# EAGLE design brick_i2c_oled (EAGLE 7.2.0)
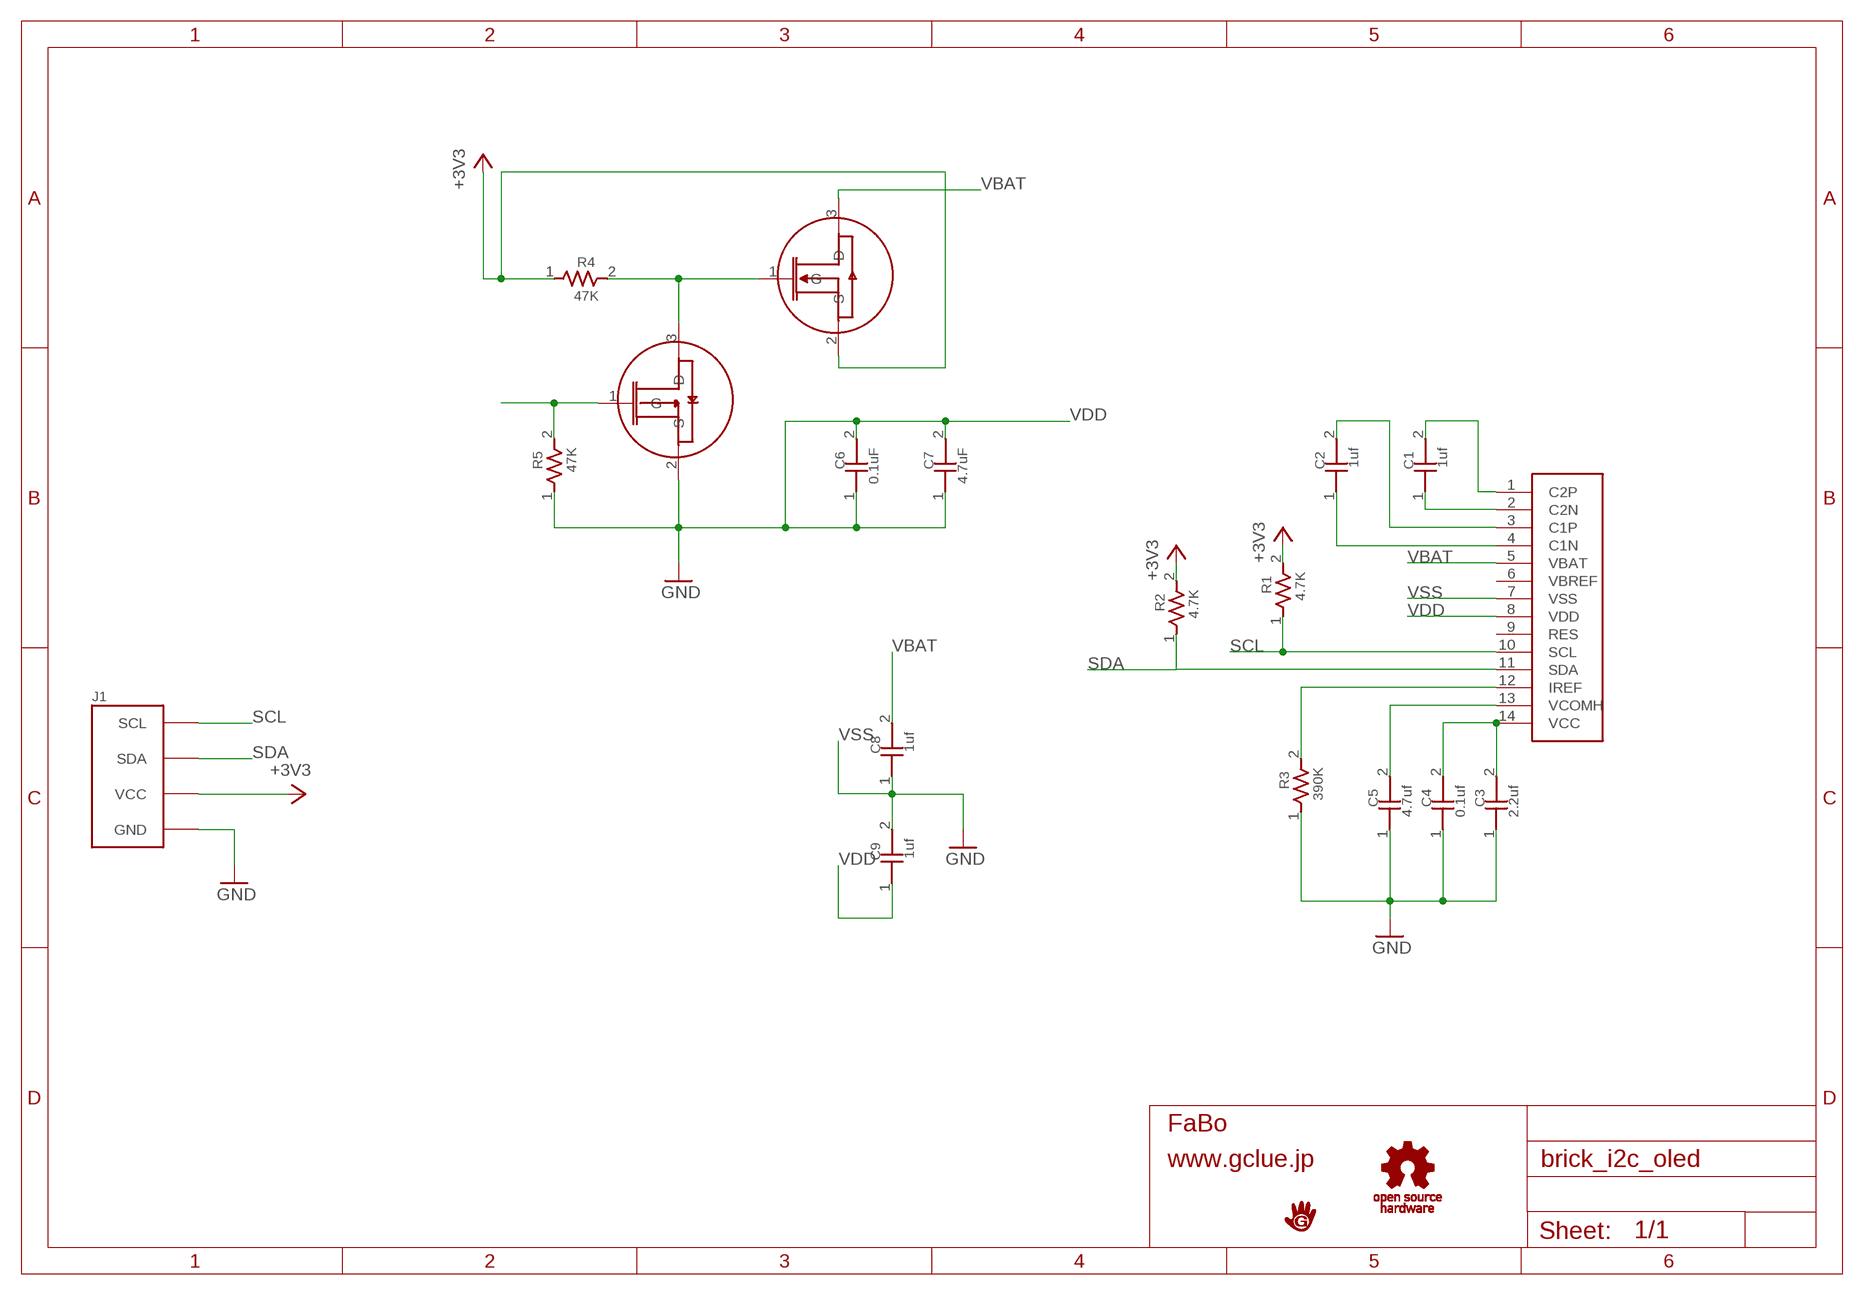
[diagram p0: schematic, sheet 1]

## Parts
C1  1uf  CAPACITOR0603  [0603]
C2  1uf  CAPACITOR0603  [0603]
C3  2.2uf  CAPACITOR0603  [0603]
C4  0.1uf  CAPACITOR0603  [0603]
C5  4.7uf  CAPACITOR0603  [0603]
C6  0.1uF  CAPACITOR0603  [0603]
C7  4.7uF  CAPACITOR0603  [0603]
C8  1uf  CAPACITOR0603  [0603]
C9  1uf  CAPACITOR0603  [0603]
J1  BRICK_I2C  [BRICK_I2C]
R1  4.7K  RESISTOR0603  [0603]
R2  4.7K  RESISTOR0603  [0603]
R3  390K  RESISTOR0603  [0603]
R4  47K  RESISTOR0603  [0603]
R5  47K  RESISTOR0603  [0603]
U$1  LOGO_GCLUE-M  [LOGO_GCLUE_M]
U$2  EASTRISING-ER-OLED0.49-1  [EASTRISING-ER-OLED0.49-1]
U$4  FAIRCHILD-FDN335  [SOT23]
U$5  FAIRCHILD-FDN338  [SOT23]
U$6  LOGO_OSHW_T-M  [LOGO_OSHW_T_M]

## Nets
+3V3: J1.VCC R1.2 R2.2 R4.1 U$4.2(S)
GND: C3.1 C4.1 C5.1 J1.GND R3.1
N$1: C1.2 U$2.1(C2P)
N$2: C1.1 U$2.2(C2N)
N$3: C2.2 U$2.3(C1P)
N$4: C2.1 U$2.4(C1N)
N$5: R5.2 U$5.1(G)
N$6: R3.2 U$2.12(IREF)
N$7: C5.2 U$2.13(VCOMH)
N$8: R4.2 U$4.1(G) U$5.3(D)
SCL: J1.SCL R1.1 U$2.10(SCL)
SDA: J1.SDA R2.1 U$2.11(SDA)
VBAT: C8.2 U$2.5(VBAT) U$4.3(D)
VCC: C3.2 C4.2 U$2.14(VCC)
VDD: C6.1 C6.2 C7.1 C7.2 C9.1 R5.1 U$2.8(VDD) U$5.2(S) ; supply symbol labelled GND
VSS: C8.1 C9.2 U$2.7(VSS) ; supply symbol labelled GND
Unconnected: U$2.6(VBREF) U$2.9(RES)

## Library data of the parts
C1-C9 = GClue-Capacitor:CAPACITOR
J1 = gclue:BRICK_I2C: FaBo Brick 4pin(I2C)
R1-R5 = GClue-Resistors:RESISTOR
U$1 = gclue:LOGO_GCLUE
U$2 = gclueParts:EASTRISING-ER-OLED0.49-1
U$4 = gclueParts:FAIRCHILD-FDN335
U$5 = gclueParts:FAIRCHILD-FDN338
U$6 = gclue:LOGO_OSHW_T

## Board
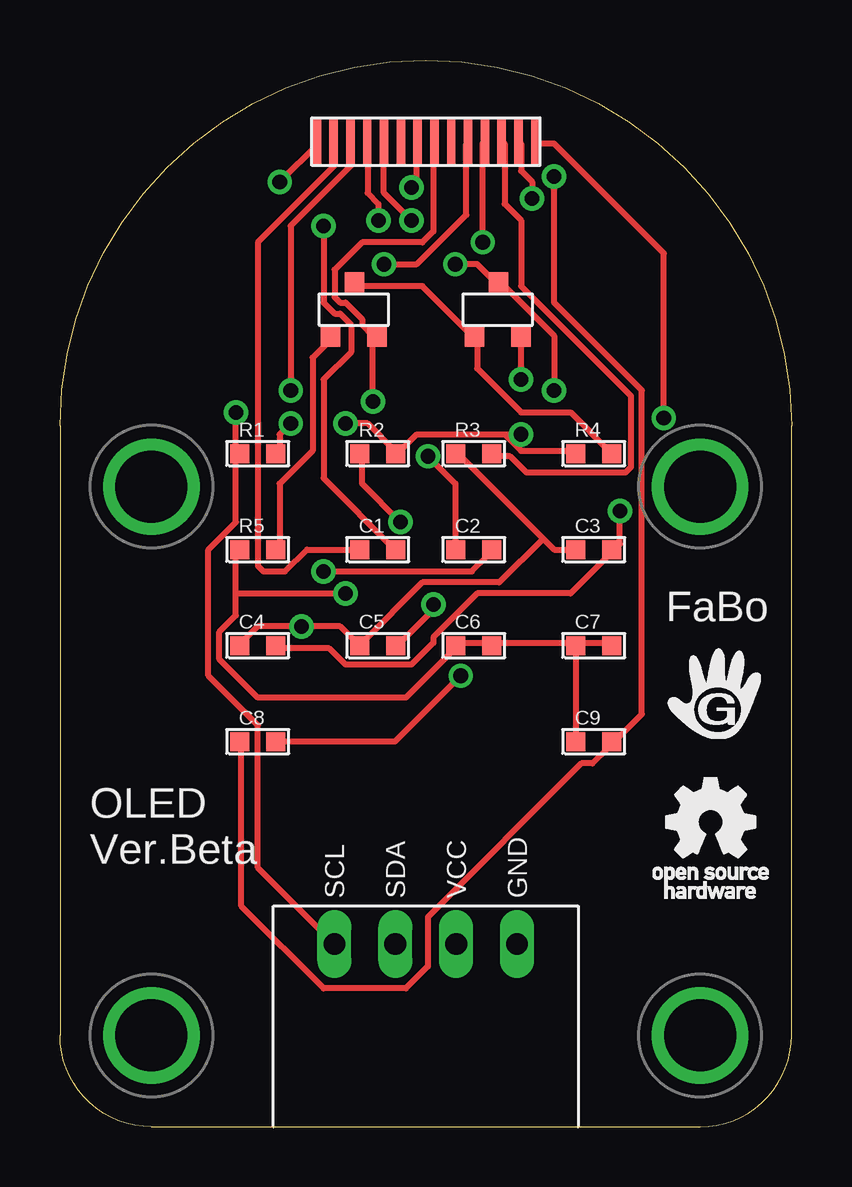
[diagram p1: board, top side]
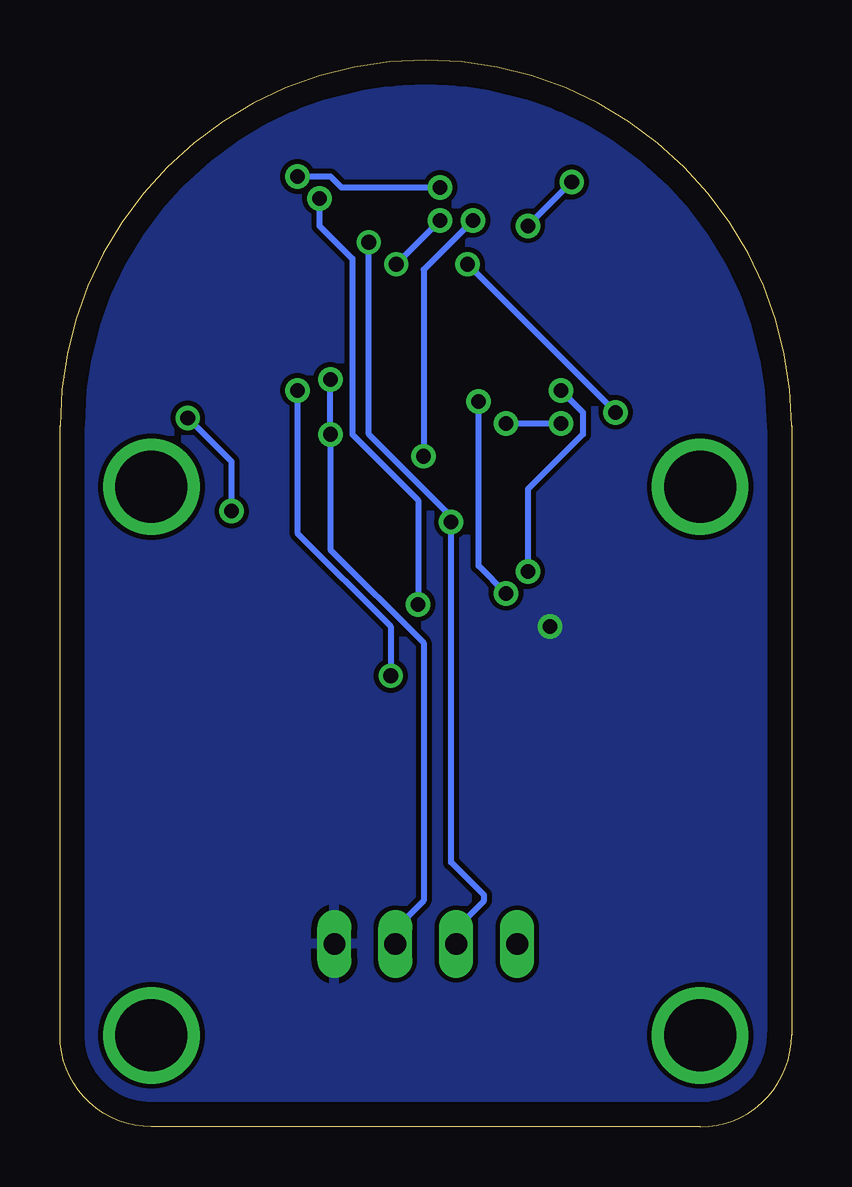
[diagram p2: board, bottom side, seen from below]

Size 30.48 x 44.45 mm. Coordinates in mm from the lower left corner, seen from the top.
Copper layers (1*16): Top 0.035mm / dielectric 1.5mm / Bottom 0.035mm
Design rules "default": minimum track width 10mil, minimum drill 24mil, track to track 8mil, track to pad 8mil, pad to pad 8mil, via to via 8mil, smd to smd 8mil, copper to edge 40mil, drill to drill 8mil, minimum pad ring 10mil, minimum via ring 8mil, stop-mask expansion 4mil, vias tented up to drill 0mil, thermal gap 10mil

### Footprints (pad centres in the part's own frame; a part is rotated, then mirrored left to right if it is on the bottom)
0603 = smd 0.8 x 0.8: 1 -0.75,0; 2 0.75,0
BRICK_I2C = drill 0.9 long: GND 3.81,-11.43; SCL -3.81,-11.43; SDA -1.27,-11.43; VCC 1.27,-11.43 | drill 3 pad 3.81: P$5 -11.43,7.62; P$6 11.43,7.62; P$7 -11.43,-15.24; P$8 11.43,-15.24
EASTRISING-ER-OLED0.49-1 = smd 0.35 x 2: 1 -4.54,0; 2 -3.84,0; 3 -3.14,0; 4 -2.44,0; 5 -1.74,0; 6 -1.04,0; 7 -0.34,0; 8 0.36,0; 9 1.06,0; 10 1.76,0; 11 2.46,0; 12 3.16,0; 13 3.86,0; 14 4.56,0
SOT23 = smd 0.8 x 0.9: 1 -0.97,-1.1; 2 0.97,-1.1; 3 0.03,1.1

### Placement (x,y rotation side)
C1  13.24,24.05 0 top
C2  17.24,24.05 0 top
C3  22.24,24.05 0 top
C4  8.24,20.05 0 top
C5  13.24,20.05 0 top
C6  17.24,20.05 0 top
C7  22.24,20.05 0 top
C8  8.24,16.05 0 top
C9  22.24,16.05 0 top
J1  15.24,19.05 0 top
R1  8.24,28.05 0 top
R2  13.24,28.05 0 top
R3  17.24,28.05 0 top
R4  22.24,28.05 0 top
R5  8.24,24.05 0 top
U$1  27.24,18.05 0 top
U$2  15.24,41.05 0 top
U$4  18.24,34.05 0 top
U$5  12.24,34.05 0 top
U$6  27.24,12.05 0 top

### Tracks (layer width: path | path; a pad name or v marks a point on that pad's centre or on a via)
+3V3  (via drill 0.61)
  Top 0.254: v9.61,29.31 9.15,28.85 9.15,28.17 R1.2 | v11.9,29.31 12.81,29.31 13.96,28.17 R2.2 14.19,28.17 14.87,28.85 18.53,28.85 | 18.53,28.85 19.21,28.17 21.27,28.17 R4.1 | v19.21,31.14 19.21,32.74 U$4.2 | 18.53,28.85 v19.21,28.85
  Bottom 0.254: v11.9,29.31 v9.61,29.31 | v19.21,31.14 v19.21,28.85 19.21,24.05 15.33,20.17 15.33,9.42 16.47,8.28 16.47,7.82 J1.VCC
GND  (via drill 0.61)
  Top 0.254: C4.1 7.56,20.17 8.24,20.85 v10.07,20.85 11.67,20.85 12.36,20.17 C5.1 12.58,20.17 15.1,22.68 18.3,22.68 20.13,24.51 | 20.13,24.51 16.7,27.94 R3.1 | 20.13,24.51 20.59,24.05 21.27,24.05 C3.1
  pour Bottom: 0.24,0.05 30.24,0.05 30.24,44.05 0.24,44.05
N$1  (via drill 0.61)
  Top 0.254: v10.98,37.54 10.98,34.34 11.44,33.88 11.67,33.88 12.13,33.43 12.13,32.28 10.98,31.14 10.98,27.03 13.96,24.05 C1.2 | v9.15,39.37 10.76,40.97 U$2.1
  Bottom 0.254: v9.15,39.37 v10.98,37.54
N$2
  Top 0.254: C1.1 12.36,24.05 10.3,24.05 9.38,23.14 8.47,23.14 8.24,23.37 8.24,36.86 11.44,40.06 11.44,40.97 U$2.2
N$3  (via drill 0.61)
  Top 0.254: v10.98,23.14 17.16,23.14 17.84,23.82 C2.2 | v9.61,30.68 9.61,37.54 12.13,40.06 12.13,40.97 U$2.3
  Bottom 0.254: v10.98,23.14 10.98,26.57 8.7,28.85 8.7,29.77 v9.61,30.68
N$4  (via drill 0.61)
  Top 0.254: v15.33,27.94 16.47,26.8 16.47,24.05 C2.1 | v13.27,37.77 13.27,38.45 12.81,38.91 12.81,40.97 U$2.4
  Bottom 0.254: v15.33,27.94 15.33,35.71 v13.27,37.77
N$5
  Top 0.254: R5.2 9.15,24.05 9.15,26.8 10.53,28.17 10.53,32.05 11.21,32.74 U$5.1
N$6
  Top 0.254: R3.2 18.07,27.94 18.76,27.94 19.44,27.25 23.56,27.25 23.79,27.48 23.79,30.45 19.21,35.03 19.21,37.77 18.53,38.45 18.53,40.97 U$2.12
N$7  (via drill 0.61)
  Top 0.254: v15.56,21.77 15.56,21.54 14.19,20.17 C5.2 | v19.67,38.68 19.67,39.37 19.21,39.83 19.21,40.97 U$2.13
  Bottom 0.254: v15.56,21.77 15.56,26.11 18.3,28.85 18.3,36.17 19.67,37.54 v19.67,38.68
N$8
  Top 0.254: R4.2 22.87,28.17 21.27,29.77 19.21,29.77 17.38,31.6 17.38,32.74 U$4.1 17.16,32.97 15.1,35.03 12.36,35.03 U$5.3
SCL  (via drill 0.61)
  Top 0.254: J1.SCL 11.21,7.82 8.24,10.79 8.24,16.74 6.18,18.8 6.18,24.05 7.33,25.2 7.33,27.94 R1.1 7.33,28.17 v7.33,29.77 | v13.5,35.94 14.87,35.94 16.93,38 16.93,40.97 U$2.10
  Bottom 0.254: v7.33,29.77 v13.5,35.94
SDA  (via drill 0.61)
  Top 0.254: v14.19,25.2 12.58,26.8 12.58,27.94 R2.1 | v17.61,36.86 17.61,40.97 U$2.11
  Bottom 0.254: J1.SDA 13.96,7.82 13.96,8.28 12.81,9.42 12.81,9.65 14.19,11.02 v14.19,25.2 14.19,25.43 17.61,28.85 v17.61,36.86
VBAT  (via drill 0.61)
  Top 0.254: v16.7,18.8 13.96,16.05 9.15,16.05 C8.2 | v20.59,30.68 20.59,32.97 18.3,35.25 U$4.3 18.07,35.25 17.38,35.94 v16.47,35.94 | v14.64,37.77 13.5,38.91 13.5,40.97 U$2.5
  Bottom 0.254: v16.7,18.8 16.7,20.85 20.59,24.74 v20.59,30.68 | v16.47,35.94 v14.64,37.77
VCC  (via drill 0.61)
  Top 0.254: C4.2 9.15,19.94 11.21,19.94 11.9,19.25 14.64,19.25 15.56,20.17 15.56,20.39 17.38,22.22 21.27,22.22 22.87,23.82 C3.2 23.1,24.05 23.33,24.28 v23.33,25.65 | v25.16,29.54 25.16,36.4 20.59,40.97 19.9,40.97 U$2.14
  Bottom 0.254: v25.16,29.54 23.33,27.71 v23.33,25.65
VDD  (via drill 0.61)
  Top 0.254: U$2.8 15.56,40.97 15.56,37.31 15.1,36.86 12.58,36.86 11.44,35.71 11.44,34.57 11.67,34.34 11.9,34.34 12.58,33.65 12.58,33.43 13.04,32.97 U$5.2 13.04,32.74 v13.04,30.23 | C9.1 21.5,19.94 C7.1 | C7.2 22.87,20.17 21.5,20.17 C7.1 | 7.33,22.22 7.33,21.31 6.64,20.62 6.64,19.48 8.24,17.88 14.41,17.88 16.47,19.94 C6.1 16.7,20.17 17.84,20.17 C6.2 18.07,20.17 21.27,20.17 C7.1 | 7.33,22.22 7.33,23.82 R5.1 | 7.33,22.22 v11.9,22.22
  Bottom 0.254: v13.04,30.23 13.04,23.37 v11.9,22.22
VSS  (via drill 0.61)
  Top 0.254: C8.1 7.56,15.82 7.56,9.19 10.98,5.77 14.41,5.77 15.33,6.68 15.33,8.74 21.73,15.14 22.19,15.14 22.87,15.82 C9.2 23.1,16.05 24.24,17.2 24.24,30.68 20.59,34.34 v20.59,39.6 | v14.64,39.14 14.87,39.37 14.87,40.97 U$2.7
  Bottom 0.254: v14.64,39.14 18.76,39.14 19.21,39.6 v20.59,39.6

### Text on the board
tPlace: FaBo | OLED / Ver.Beta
